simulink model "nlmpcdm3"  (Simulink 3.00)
settings: Solver=ode45  SolverMode=SingleTasking  StartTime=0.0  StopTime=30  FixedStep=[]  MaxStep=1  RelTol=1e-3  AbsTol=1e-3
PreLoadFcn:
  | demo2dat
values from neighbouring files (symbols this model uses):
  d0 = []    [demo1dat.m]    (also in demo2dat.m = 0; essai1dat.m)
  dmodel = []    [demo1dat.m]    (also in essai1dat.m; essai2dat.m; mynlcmpc.m = modelpd(:,nu+1:nund); mynlcmpc2.m = modelpd(:,nu+1:nund))
  m = 4    [demo1dat.m]    (also in demo2dat.m = 3; essai1dat.m; essai2dat.m = 6; mynlcmpc.m = mp(1:max(size(mp))-1))
  model = tfd2step(1.6,delt,1,g)    [essai2dat.m]    (also in mynlcmpc.m = modelpd(:,1:nu); mynlcmpc2.m = modelpd(:,1:nu); mynlcmpc3.m = modelpd(:,1:nu); scrtp1.m = tfd2step(tfinal,Ts,1,g))
  p = 10    [demo1dat.m]    (also in demo2dat.m; essai1dat.m; essai2dat.m; mynlcmpc.m = mp(max(size(mp))))
  r = [68.3 2]    [demo1dat.m]    (also in demo2dat.m = [0 0 0]; essai1dat.m; essai2dat.m = 10; mynlcmpc.m = zeros(1,ny))
  u0 = [100 1]    [demo1dat.m]    (also in demo2dat.m = [0 0]; essai1dat.m; pmnonl.m = zeros(3,1))
  u_lim = [100 1 200 3 200 200]    [demo1dat.m]    (also in demo2dat.m = [-10*[1 1] 10*[1 1] 2*[1 1]]; essai1dat.m)
  uwt = [0 0]    [demo1dat.m]    (also in demo2dat.m = 0.6*[1 1]; essai1dat.m; essai2dat.m = 1; mynlcmpc.m = ryuwt(:,2*ny+1:2*ny+nu))
  y_lim = [-inf -inf inf inf]    [demo1dat.m]    (also in demo2dat.m = [-inf -inf -inf inf inf inf]; essai1dat.m)
  ywt = [1 1]    [demo1dat.m]    (also in demo2dat.m = [0.2,0,1]; essai1dat.m; essai2dat.m = 1; mynlcmpc.m = ryuwt(:,ny+1:2*ny))
libraries: nlmpclib x1

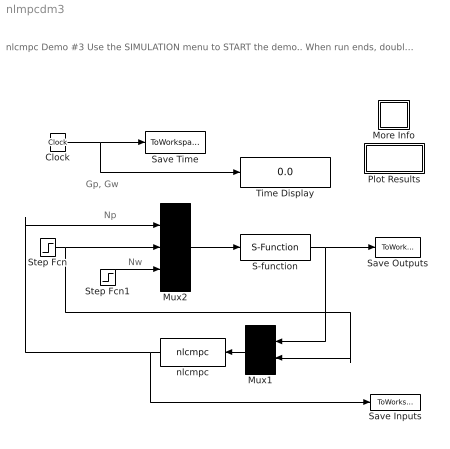
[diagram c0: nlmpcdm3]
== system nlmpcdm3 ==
  note: nlcmpc Demo #3 Use the SIMULATION menu to START the demo.. When run ends, double click on PLOT RESULTS. (Double click on the "?" for more info)
  note: Nw
  note: Np
  note: Gp, Gw
  Clock : Clock
  More Info : Subsystem
  Mux1 : Mux  Orientation=left  Inputs=[3 1]
  Mux2 : Mux  Inputs=[2 1 1]
  Plot Results : Subsystem
  S-function : S-Function  FunctionName=papmach  PortCounts=[]  SFunctionModules=''
  Save Inputs : ToWorkspace  VariableName=u  SampleTime=0
  Save Outputs : ToWorkspace  VariableName=y  SampleTime=0
  Save Time : ToWorkspace  VariableName=t  SampleTime=0
  Step Fcn : Step  Time=0  Before=0  After=1  SampleTime=0
  Step Fcn1 : Step  Time=0  Before=0  After=0  SampleTime=0
  Time Display : Display
  nlcmpc : nlmpclib/nlcmpc  Orientation=left  modelpd=[model dmodel]  ryuwt=[r ywt uwt]  mp=[m p]  yulim=[y_lim u_lim]  tfilter=tfilter  ud0=[u0 d0]
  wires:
  Clock/1 -> Save Time/1, Time Display/1
  S-function/1 -> Mux1/1, Save Outputs/1
  Step Fcn/1 -> Mux2/2, Mux1/2
  Step Fcn1/1 -> Mux2/3
  Mux2/1 -> S-function/1
  nlcmpc/1 -> Save Inputs/1, Mux2/1
  Mux1/1 -> nlcmpc/1

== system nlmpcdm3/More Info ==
  note: Use the Simulation menu to Start the demo. At the end of the simulation, double-click on "Plot Results" to have inputs and outputs displayed in a figure window using the MPC Tools PLOTEACH command.
  note: This demonstration shows the use of nlcmpc. The plant is the paper machine headbox discussed in Section 3.4 of the manual. See nlcmpc in Command Reference for details.

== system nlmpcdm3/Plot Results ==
